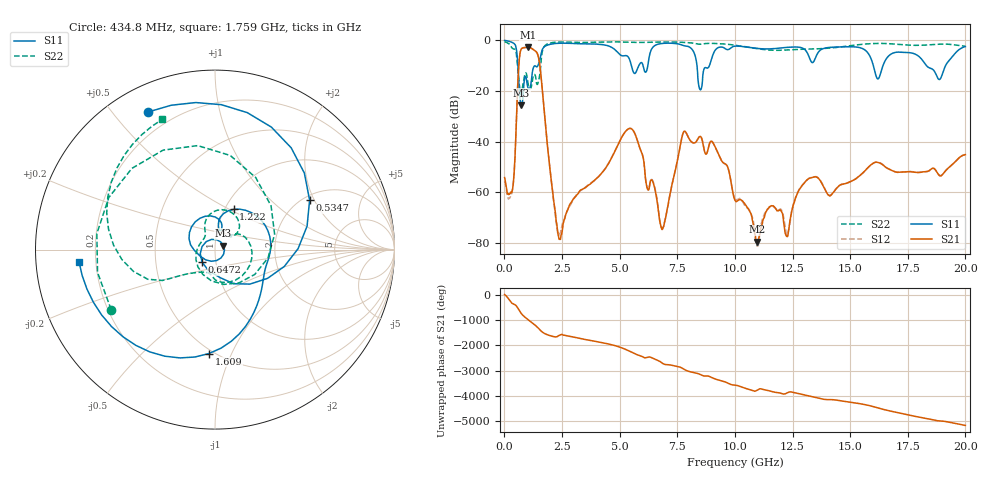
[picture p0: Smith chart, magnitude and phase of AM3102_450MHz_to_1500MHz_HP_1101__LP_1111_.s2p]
!Agilent Technologies,E8364B,MY43040894,A.07.50.67
!Agilent E8364B: A.07.50.67
!Date: Thursday, January 11, 2018 06:41:15
!Correction: S11(Full 2 Port(1,2))
!S21(Full 2 Port(1,2))
!S12(Full 2 Port(1,2))
!S22(Full 2 Port(1,2))
!S2P File: Measurements: S11, S21, S12, S22:
# Hz S  dB  R 50
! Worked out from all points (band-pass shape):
!   1601 points, 10 MHz to 20 GHz, reference 50 ohm
!   highest |S21| = -2.78 dB at 1.034 GHz (marker M1); lowest = -79.5 dB at 10.95 GHz (marker M2)
!   |S21| within 3 dB of the highest: 668.4 MHz to 1.452 GHz (783.2 MHz wide, 73.9 % of centre)
!   lowest |S11| = -25.6 dB at 734.6 MHz (marker M3), VSWR 1.11, Z = 54.9 + j2.51 ohm
!   |S11| at or under -10 dB: 588.1 MHz to 1.454 GHz (865.8 MHz wide, 84.8 % of centre); 8.356 GHz to 8.895 GHz (539.2 MHz wide, 6.25 % of centre); 18.31 GHz to 19.14 GHz (827.9 MHz wide, 4.42 % of centre)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
!   |S22| runs from -21.3 to -0.5 dB; largest |S21 - S12| = 0.00071
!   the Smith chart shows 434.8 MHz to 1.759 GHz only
!   S11 on the Smith chart (normalised r, x): 434.8 MHz: 0.11, +0.62; 534.7 MHz: 2.16, +1.84; 647.2 MHz: 0.86, -0.12; 1.222 GHz: 1.10, +0.53; 1.609 GHz: 0.47, -0.82; 1.759 GHz: 0.14, -0.04
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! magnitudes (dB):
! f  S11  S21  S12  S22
! 10 MHz  -0.1  -54.2  -55.8  -0.5
! 434.8 MHz  -1.4  -50.7  -50.6  -3.5
! 534.7 MHz  -4.5  -27.7  -27.7  -6.7
! 647.2 MHz  -20.0  -7.5  -7.5  -17.4
! 734.6 MHz  -25.6  -3.4  -3.4  -21.0
! 1.034 GHz  -19.0  -2.8  -2.8  -17.5
! 1.222 GHz  -12.1  -3.4  -3.4  -15.5
! 1.609 GHz  -4.7  -15.9  -15.9  -6.6
! 1.759 GHz  -2.4  -31.3  -31.3  -2.1
! 2.384 GHz  -1.2  -78.6  -76.9  -0.7
! 3.346 GHz  -1.4  -59.0  -59.0  -0.9
! 5.47 GHz  -8.6  -34.8  -34.8  -0.8
! 6.682 GHz  -1.5  -67.4  -66.6  -0.7
! 6.932 GHz  -1.2  -72.6  -72.2  -0.7
! 7.819 GHz  -2.2  -35.9  -35.9  -0.9
! 8.493 GHz  -19.5  -37.9  -37.9  -1.6
! 10.01 GHz  -2.3  -63.2  -62.7  -2.0
! 10.95 GHz  -3.2  -79.5  -81.1  -3.3
! 13.34 GHz  -8.7  -54.2  -54.1  -3.4
! 16.68 GHz  -6.1  -50.8  -50.8  -1.3
! 18.86 GHz  -15.5  -53.3  -53.2  -1.5
! 20 GHz  -2.5  -45.1  -45.1  -2.4
